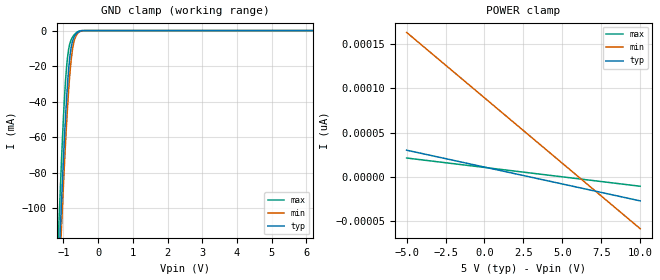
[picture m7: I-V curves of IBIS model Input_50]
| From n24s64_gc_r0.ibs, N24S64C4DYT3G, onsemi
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|//////////////////////////////////////////////////////////////////////////////
|//////////////////////////////////////////////////////////////////////////////
[Model]  Input_50
Model_type Input
Vinh = 3.50
Vinl = 1.50
|  variable   typ   min   max
C_comp   6pF   6pF   6pF
|//////////////////////////////////////////////////////////////////////////////
[Temperature Range]   25   85   -40
|//////////////////////////////////////////////////////////////////////////////
[Voltage Range]   5.00V   4.50V   5.50V
|//////////////////////////////////////////////////////////////////////////////
[POWER Clamp Reference] 5.00V   4.50V   5.50V
|//////////////////////////////////////////////////////////////////////////////
[GND Clamp Reference]   0V   0V   0V
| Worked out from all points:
|   GND clamp passes 1 mA (typ) near -0.59 V on its own axis
|//////////////////////////////////////////////////////////////////////////////
[GND Clamp]
|   Voltage   I(typ)   I(min)   I(max)
-5V       -1.846A    -1.846A    -1.907A
-1.15V    -137.8mA   -152mA     -116.8mA
-1.1V     -115.6mA   -130mA     -93.58mA
-1.075V   -104.5mA   -119mA     -81.5mA
-1.05V    -93.42mA   -108mA     -69.87mA
-950mV    -52.01mA   -66.64mA   -31mA
-900mV    -35.04mA   -48.68mA   -18.18mA
-825mV    -16.36mA   -26.6mA    -8.031mA
-725mV    -5.098mA   -8.814mA   -3.265mA
-650mV    -2.141mA   -3.47mA    -1.543mA
-550mV    -529uA     -840uA     -262uA
10V       30.37pA    170.5pA    20.47pA
|//////////////////////////////////////////////////////////////////////////////
[POWER Clamp]
|   Voltage   I(typ)   I(min)   I(max)
-5V       30.37pA    163.2pA    21.53pA
0V        11.32pA    89.4pA     10.92pA
5V        -7.731pA   15.64pA    314.7fA
10V       -26.78pA   -58.12pA   -10.29pA
